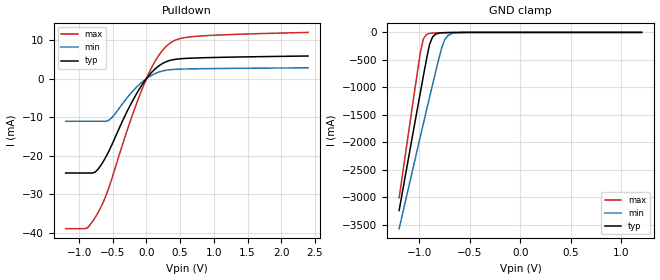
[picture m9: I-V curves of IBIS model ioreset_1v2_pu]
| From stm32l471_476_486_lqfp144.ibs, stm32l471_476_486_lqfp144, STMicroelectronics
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|   Model ioreset_1v2_pu
[Model]  ioreset_1v2_pu
Model_type I/O_open_drain
Polarity   Inverting
Enable   Active-High
Vinl =   0.360000V
Vinh =   0.840000V
Vmeas =  0.600000V
Cref =   100.000000nF
Rref =   1.000000k
Vref =   1.200000V
C_comp   0.478720pF   0.386870pF   0.488870pF
[Temperature Range]   25.000000   0.125000k   -40.000000
[Pullup Reference]   1.200000V   1.080000V   1.320000V
[Pulldown Reference]   0.0V   0.0V   0.0V
[POWER Clamp Reference]   1.200000V   1.080000V   1.320000V
[GND Clamp Reference]   0.0V   0.0V   0.0V
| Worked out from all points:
|   slope of the pulldown table from 0 to 0.18 V, typ, clamps not added: 55.7 ohm
|   GND clamp passes 1 mA (typ) near -0.60 V on its own axis
[Pulldown]
|Voltage   I(typ)   I(min)   I(max)
-1.2V     -24.47mA   -11.06mA   -38.87mA
-880mV    -24.47mA   -11.06mA   -38.7mA
-720mV    -23.49mA   -11.06mA   -34.76mA
-600mV    -20.22mA   -11.06mA   -30.25mA
-520mV    -17.39mA   -10.23mA   -26.24mA
-240mV    -6.868mA   -3.965mA   -11.02mA
-40mV     -966.2uA   -522.8uA   -1.659mA
120mV     2.364mA    1.225mA    4.26mA
320mV     4.547mA    2.231mA    8.763mA
480mV     5.089mA    2.429mA    10.27mA
720mV     5.323mA    2.523mA    10.91mA
2.4V      5.843mA    2.784mA    11.96mA
[GND_clamp]
|Voltage   I(typ)   I(min)   I(max)
-1.2V     -3.237A    -3.567A    -3.007A
-990mV    -1.09A     -1.891A    -366.7mA
-960mV    -790.4mA   -1.655A    -117.3mA
-930mV    -495.2mA   -1.419A    -39.03mA
-900mV    -224mA     -1.186A    -17.33mA
-870mV    -83.94mA   -954.7mA   -11.02mA
-780mV    -7.786mA   -289.5mA   -5.907mA
-750mV    -4.95mA    -134.8mA   -4.824mA
-720mV    -3.507mA   -62.23mA   -3.833mA
-660mV    -1.911mA   -14.46mA   -2.15mA
-540mV    -364.7uA   -1.228mA   -309.9uA
1.2V      0A         0A         0A
[POWER_clamp]
|Voltage   I(typ)   I(min)   I(max)
-1.2V     0A         0A         0A
0V        0A         0A         0A
[Ramp]
| variable   typ   min   max
dV/dt_r  0.71922/0.66867u   0.64662/0.60089u   0.79151/0.60032u
dV/dt_f  0.71922/37.98593n   0.64662/77.79078n   0.79151/22.11929n
R_load = 40.000000k
